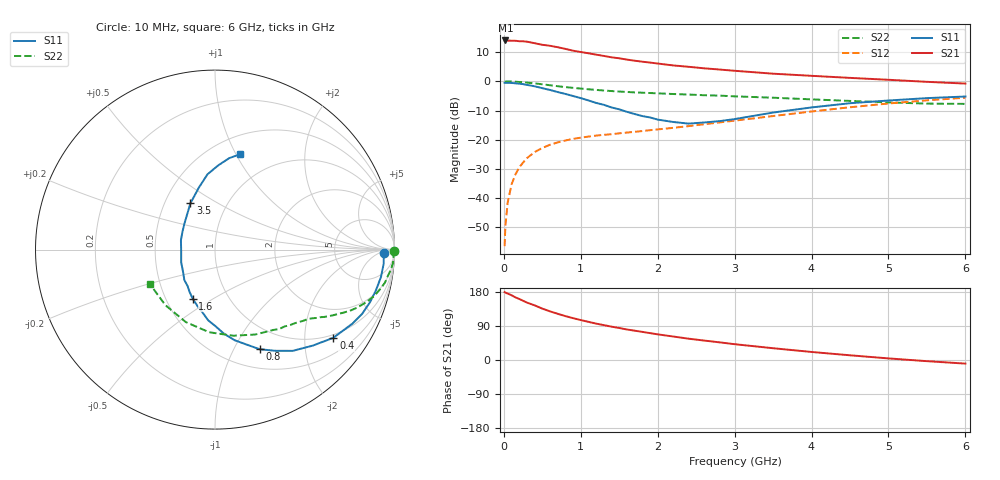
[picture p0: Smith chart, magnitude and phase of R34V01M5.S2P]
! SIEMENS Small Signal Semiconductors
! BFR181
! Si NPN RF Bipolar Junction Transistor in SOT23
! VCE = 4 V  IC = 1.5 mA
! Common Emitter S-Parameters:  May  1996
# GHz  S  MA  R  50
!  f  S11  S21  S12  S22
! GHz  MAG  ANG  MAG  ANG  MAG  ANG  MAG  ANG
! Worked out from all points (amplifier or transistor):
!   36 points, 10 MHz to 6 GHz, reference 50 ohm
!   highest |S21| = 14.0 dB at 20 MHz (marker M1)
!   |S21| within 3 dB of that: start of sweep to 817 MHz
!   unconditionally stable (mu >= 1): 1.769 GHz to 3.543 GHz
!   at 250 MHz: K = 0.19, MSG = 20.8 dB, |S12| = -27.8 dB
!   at 1.4 GHz: K = 0.88, MSG = 13.2 dB, |S12| = -18.1 dB
!   at 6 GHz: K = 0.86, MSG = 2.4 dB, |S12| = -5.6 dB
!   S11 on the Smith chart (normalised r, x): 10 MHz: 32, -10; 400 MHz: 0.91, -2.75; 800 MHz: 0.72, -1.27; 1.6 GHz: 0.68, -0.41; 3.5 GHz: 0.67, +0.38; 6 GHz: 0.68, +1.04
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0.01  0.9441 -1.0  4.981 179.2  0.0015 88.1  0.9971 -0.5
0.02  0.9409 -2.1  5.011 177.9  0.0033 84.5  0.9907 -0.9
0.05  0.9433 -4.7  4.982 175.3  0.0084 87.1  0.9955 -2.3
0.1  0.9371 -9.5  4.958 170.9  0.0171 84.6  0.994 -4.5
0.15  0.9243 -14.4  4.949 165.3  0.0253 80.4  0.984 -6.9
0.3  0.8697 -28.3  4.776 151.5  0.0483 73.0  0.9501 -13.0
0.4  0.8223 -36.7  4.496 144.2  0.0613 68.1  0.9226 -16.4
0.5  0.7633 -44.5  4.224 135.6  0.0722 64.0  0.8892 -19.4
0.6  0.7111 -52.5  4.063 128.4  0.0818 60.6  0.8569 -22.1
0.7  0.655 -59.4  3.839 121.9  0.09 57.6  0.8252 -24.4
0.8  0.6078 -65.9  3.59 115.8  0.0969 55.0  0.7963 -26.2
0.9  0.56 -71.3  3.347 110.4  0.1033 53.6  0.7726 -27.7
1.1  0.4704 -84.0  3.022 100.7  0.1131 51.0  0.7307 -30.6
1.3  0.396 -95.5  2.72 92.0  0.1212 49.8  0.6954 -32.8
1.6  0.3 -114.5  2.355 80.5  0.1325 49.8  0.6571 -35.8
1.9  0.2406 -135.3  2.096 70.9  0.1454 50.7  0.6302 -39.1
2.2  0.2013 -159.4  1.873 62.0  0.1596 51.9  0.606 -42.5
2.8  0.2076 150.6  1.593 46.7  0.1972 53.6  0.5691 -51.0
3.5  0.2919 118.0  1.351 31.1  0.2542 52.8  0.5238 -64.6
4.5  0.4216 95.7  1.145 12.4  0.3595 46.1  0.4616 -94.0
5.5  0.5155 81.2  0.98 -3.1  0.4725 33.7  0.415 -131.7
6  0.5491 75.3  0.915 -9.5  0.5239 26.3  0.4106 -152.2
